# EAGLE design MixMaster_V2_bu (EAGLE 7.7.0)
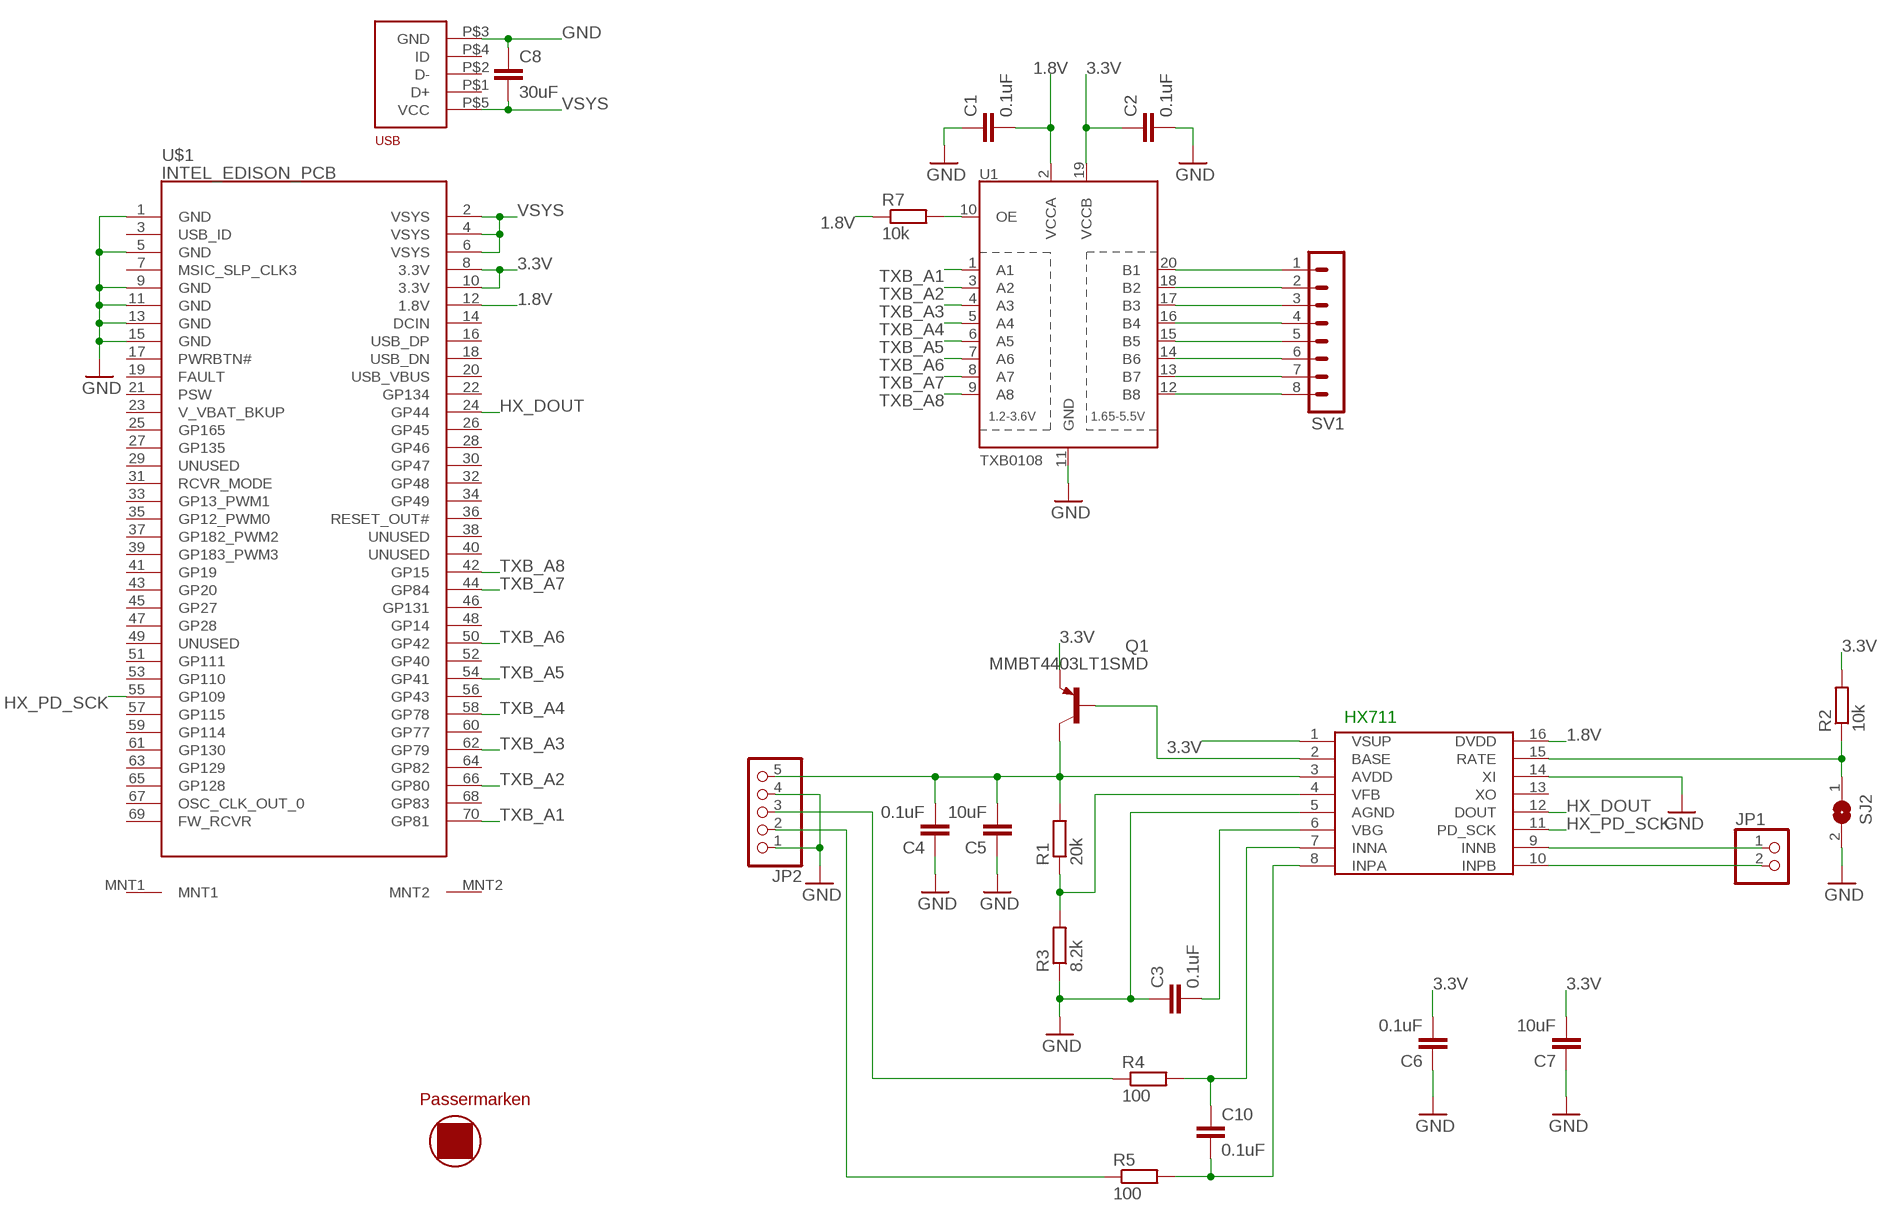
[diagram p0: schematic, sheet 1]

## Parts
C1  0.1uF  C-EUC0805  [C0805]
C2  0.1uF  C-EUC0805  [C0805]
C3  0.1uF  C-EUC0805  [C0805]
C4  0.1uF  C-EUC0805  [C0805]
C5  10uF  C-EUC0805  [C0805]
C6  0.1uF  C-EUC0805  [C0805]
C7  10uF  C-EUC0805  [C0805]
C8  30uF  C-EUC0805  [C0805]
C10  0.1uF  C-EUC0805  [C0805]
JP1  PINHD-1X2  [1X02]
JP2  PINHD-1X5  [1X05]
Q1  MMBT4403LT1SMD  [SOT23-BEC]
R1  20k  R-EU_R0805  [R0805]
R2  10k  R-EU_R0805  [R0805]
R3  8.2k  R-EU_R0805  [R0805]
R4  100  R-EU_R0805  [R0805]
R5  100  R-EU_R0805  [R0805]
R7  10k  R-EU_R0805  [R0805]
SJ2  SJ  [SJ]
SV1  MA08-1  [MA08-1]
U1  TXB0108  [TSSOP20]
U$1  INTEL_EDISON_PCB  [INTEL_EDISON]
U$2  HX711  [SO16]
U$3  USB  [USB]
U$4  PASSERMARKEN  [MASTERSUBSTRAT-MITPASSERMARKEN]

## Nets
1.8V: C1.2 R7.1 U1.2(VCCA) U$1.12(1.8V) U$2.16(DVDD)
3.3V: C2.1 C6.2 C7.2 Q1.E R2.2 U1.19(VCCB) U$1.8(3.3V) U$1.10(3.3V) U$2.1(VSUP)
GND: C1.1 C2.2 C3.1 C4.1 C5.1 C6.1 C7.1 C8.1 JP2.1 JP2.4 R3.1 SJ2.2 U1.11(GND) U$1.1(GND) U$1.5(GND) U$1.9(GND) U$1.11(GND) U$1.13(GND) U$1.15(GND) U$2.5(AGND) U$2.14(XI) U$3.P$3(GND)
HX_DOUT: U$1.24(GP44) U$2.12(DOUT)
HX_PD_SCK: U$1.55(GP109) U$2.11(PD_SCK)
N$1: R7.2 U1.10(OE)
N$2: SV1.1 U1.20(B1)
N$5: SV1.4 U1.16(B4)
N$6: SV1.5 U1.15(B5)
N$7: SV1.6 U1.14(B6)
N$8: SV1.7 U1.13(B7)
N$9: SV1.8 U1.12(B8)
N$10: C4.2 C5.2 JP2.5 Q1.C R1.2 U$2.3(AVDD)
N$11: Q1.B U$2.2(BASE)
N$12: R2.1 SJ2.1 U$2.15(RATE)
N$13: JP1.1 U$2.9(INNB)
N$14: JP1.2 U$2.10(INPB)
N$15: R1.1 R3.2 U$2.4(VFB)
N$16: JP2.2 R5.1
N$17: C3.2 U$2.6(VBG)
N$18: C10.1 R4.2 U$2.7(INNA)
N$19: C10.2 R5.2 U$2.8(INPA)
N$20: JP2.3 R4.1
N$21: SV1.2 U1.18(B2)
N$22: SV1.3 U1.17(B3)
TXB_A1: U1.1(A1) U$1.70(GP81)
TXB_A2: U1.3(A2) U$1.66(GP80)
TXB_A3: U1.4(A3) U$1.62(GP79)
TXB_A4: U1.5(A4) U$1.58(GP78)
TXB_A5: U1.6(A5) U$1.54(GP41)
TXB_A6: U1.7(A6) U$1.50(GP42)
TXB_A7: U1.8(A7) U$1.44(GP84)
TXB_A8: U1.9(A8) U$1.42(GP15)
VSYS: C8.2 U$1.2(VSYS) U$1.4(VSYS) U$1.6(VSYS) U$3.P$5(VCC)
Unconnected: U$1.3(USB_ID) U$1.7(MSIC_SLP_CLK3) U$1.14(DCIN) U$1.16(USB_DP) U$1.17(PWRBTN#) U$1.18(USB_DN) U$1.19(FAULT) U$1.20(USB_VBUS) U$1.21(PSW) U$1.22(GP134) U$1.23(V_VBAT_BKUP) U$1.25(GP165) U$1.26(GP45) U$1.27(GP135) U$1.28(GP46) U$1.29(UNUSED) U$1.30(GP47) U$1.31(RCVR_MODE) U$1.32(GP48) U$1.33(GP13_PWM1) U$1.34(GP49) U$1.35(GP12_PWM0) U$1.36(RESET_OUT#) U$1.37(GP182_PWM2) U$1.38(UNUSED) U$1.39(GP183_PWM3) U$1.40(UNUSED) U$1.41(GP19) U$1.43(GP20) U$1.45(GP27) U$1.46(GP131) U$1.47(GP28) U$1.48(GP14) U$1.49(UNUSED) U$1.51(GP111) U$1.52(GP40) U$1.53(GP110) U$1.56(GP43) U$1.57(GP115) U$1.59(GP114) U$1.60(GP77) U$1.61(GP130) U$1.63(GP129) U$1.64(GP82) U$1.65(GP128) U$1.67(OSC_CLK_OUT_0) U$1.68(GP83) U$1.69(FW_RCVR) U$1.MNT1 U$1.MNT2 U$2.13(XO) U$3.P$1(D+) U$3.P$2(D-) U$3.P$4(ID)

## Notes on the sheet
- HX711

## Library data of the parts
C1-C8 C10 = rcl:C-EU: CAPACITOR, European symbol
JP1 = pinhead:PINHD-1X2: PIN HEADER
JP2 = pinhead:PINHD-1X5: PIN HEADER
Q1 = transistor-pnp:MMBT4403*: PNP Transistror
R1-R5 R7 = rcl:R-EU_: RESISTOR, European symbol
SJ2 = jumper:SJ: SMD solder JUMPER
SV1 = con-lstb:MA08-1: PIN HEADER; OC_FARNELL: unknown; OC_NEWARK: unknown
U1 = TXB0108:TXB0108: 8-Bit Bi-Directional Level Shifter 1.2V-3.6V (VCCA) to 1.65V-5.5V (VCCB) bi-directional level shifter with auto direction sensing. Max data rate - VCCA 1.8V: 20Mbps (50ns), VCCA 3.3V: 100Mbps (10ns) Digikey: 296-21527-1-ND; AVAILABILITY: Unavailable; DESCRIPTION: 8-Bit Bidirectional Voltage-Level Translator with Auto Direction Sensing and +/-15-kV ESD Protect; MF: Texas Instruments; MP: TXB0108; PACKAGE: None; PRICE: None
U$1 = e14_Intel_Edison_RevA:INTEL_EDISON_PCB: Intel Edison Compute Module. Ideal for creating your own PCB to host an Edison. Created for www.element14.com by Dave of Young Circuit Designs. Note: 70-pin connector on the Edison is a 1.5mm-tall Hirose plug DF40C-70DP-0.4V(51) Mating Hirose receptacle connectors of varying heights include the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
U$2 = HX711:HX711
U$3 = USB_Buchse:USB
U$4 = lmhs:PASSERMARKEN

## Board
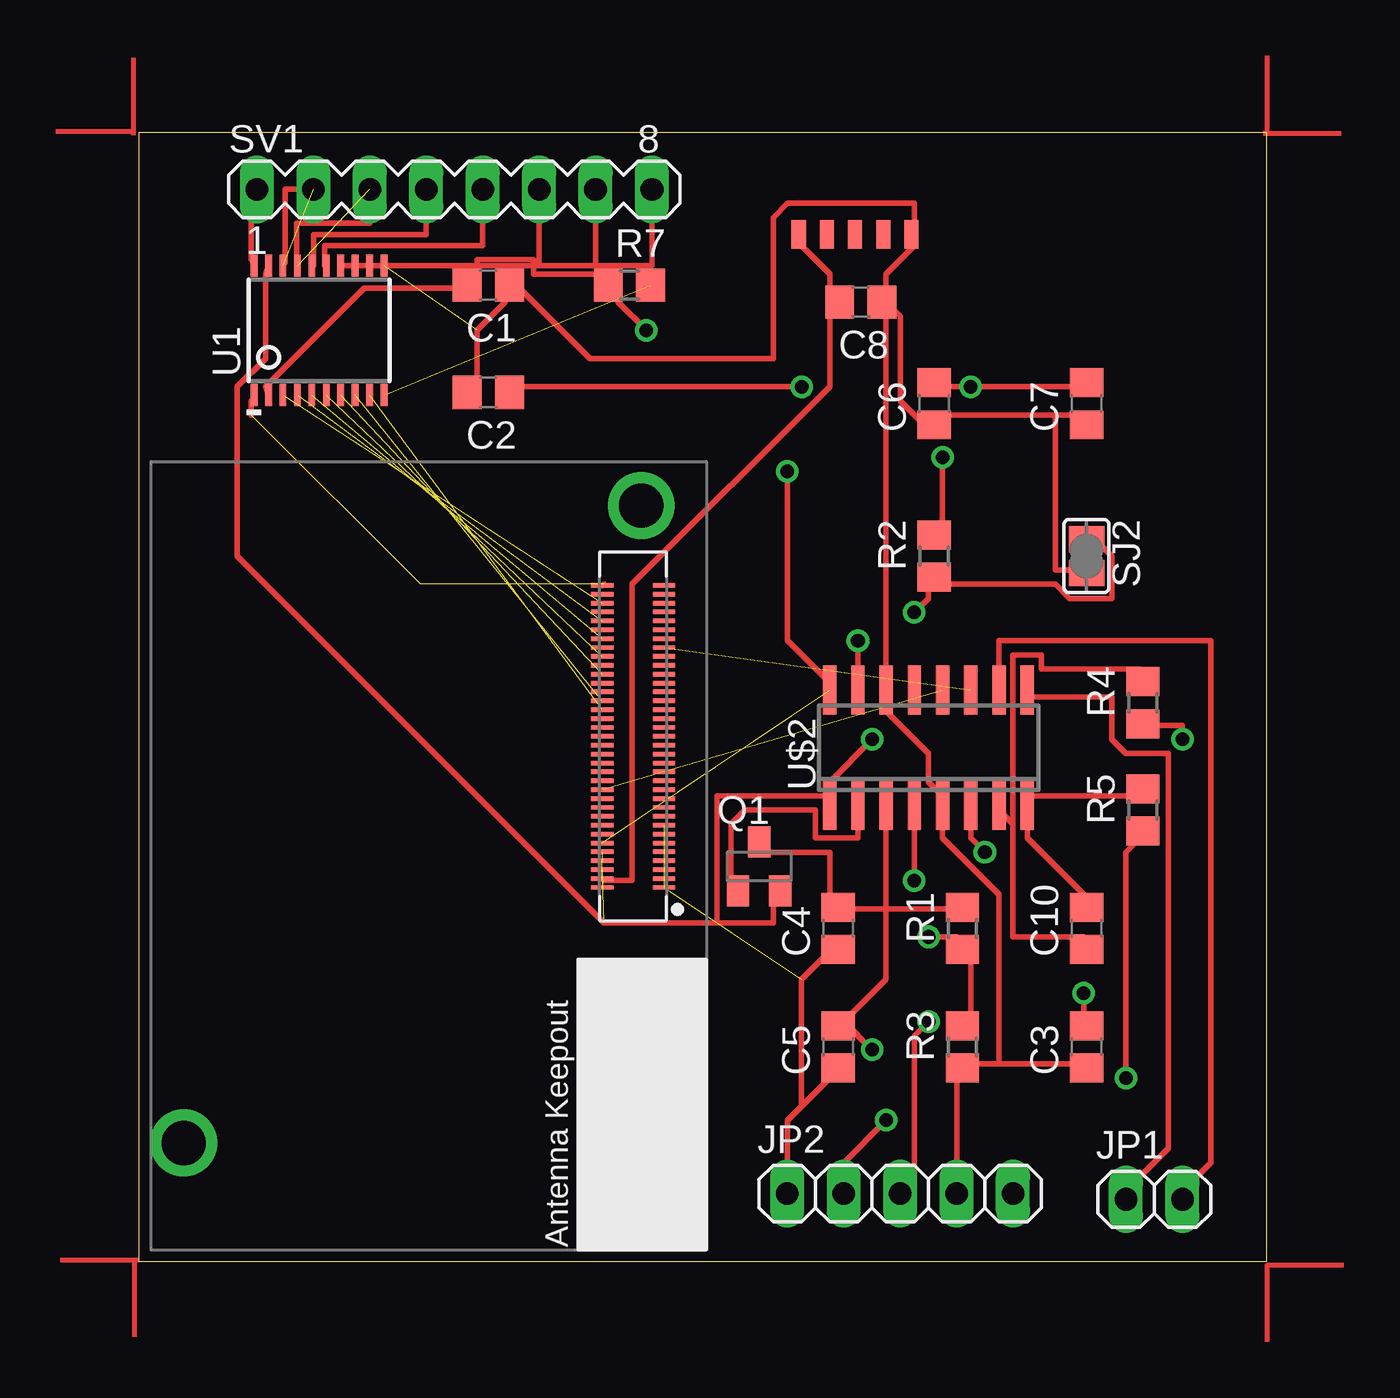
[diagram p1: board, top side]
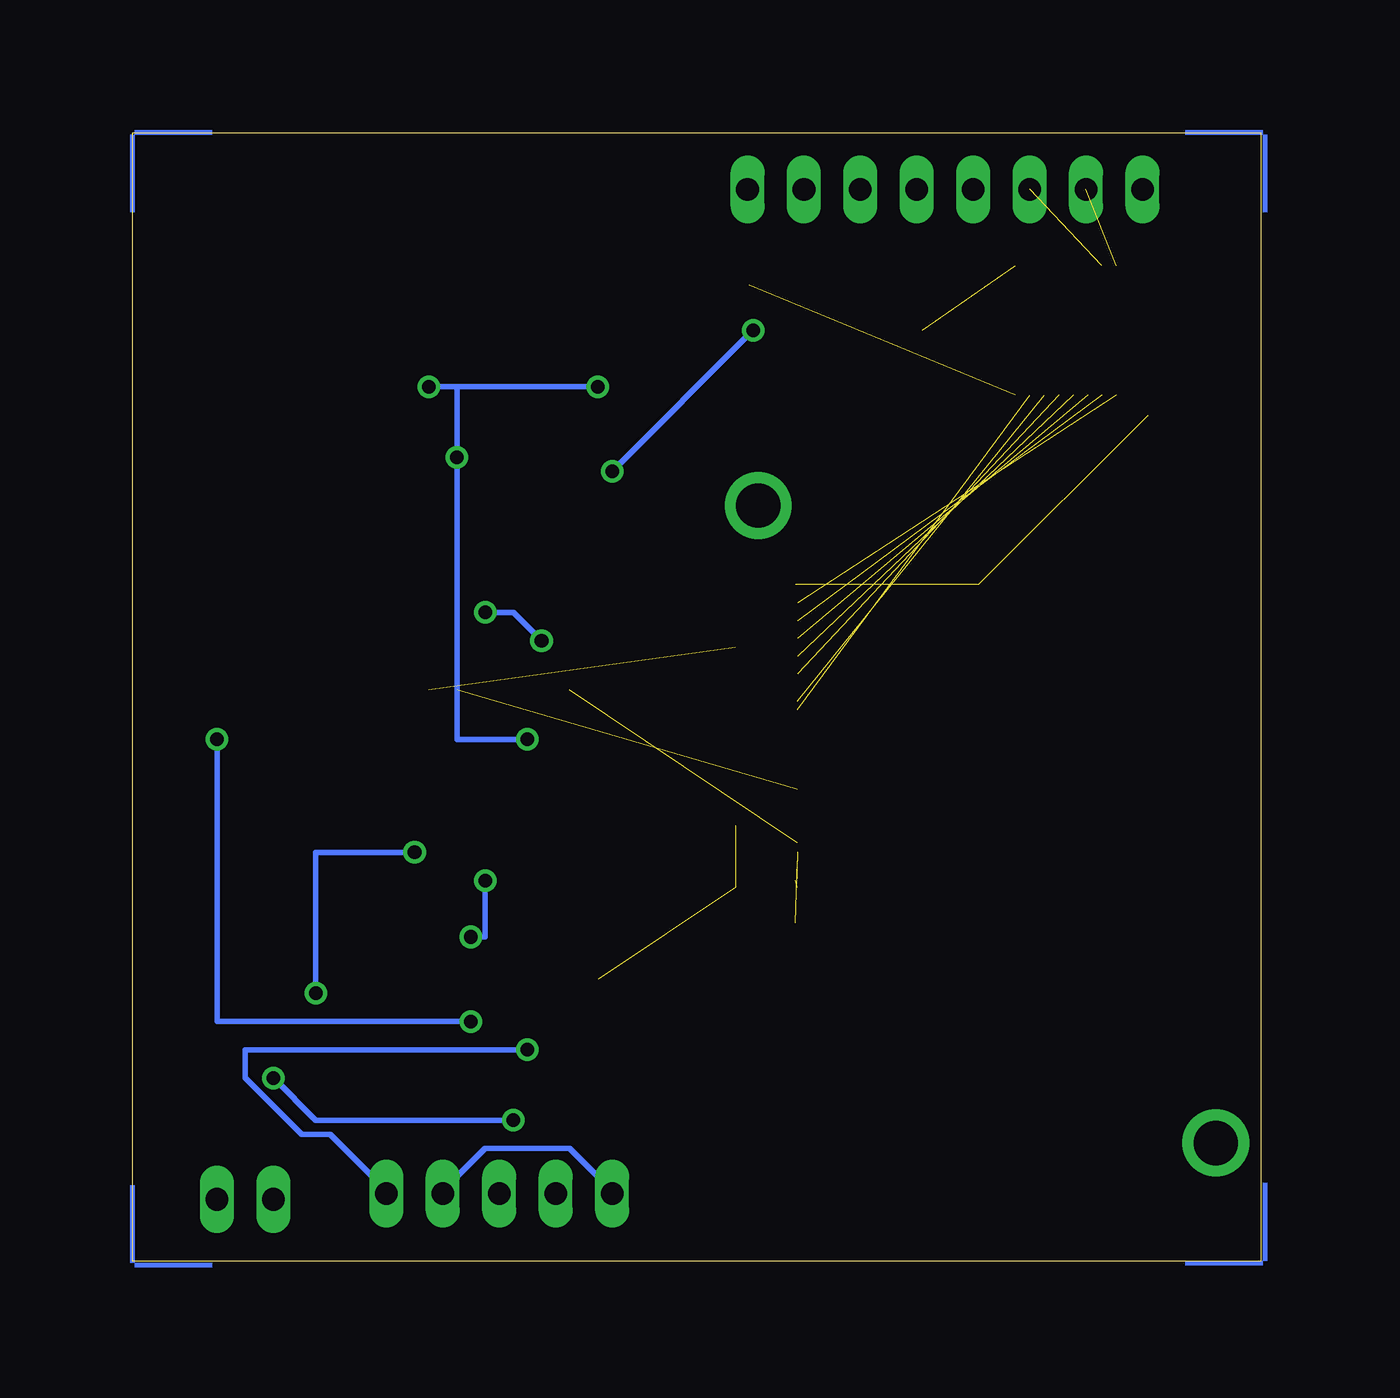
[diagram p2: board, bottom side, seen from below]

Size 50.8 x 50.8 mm. Coordinates in mm from the lower left corner, seen from the top.
Outline: 0,0 50.8,0 50.8,50.8 0,50.8 0,0
Copper layers (1*16): Top 0.035mm / dielectric 1.5mm / Bottom 0.035mm
Design rules "default": minimum track width 10mil, minimum drill 24mil, track to track 8mil, track to pad 8mil, pad to pad 8mil, via to via 8mil, smd to smd 8mil, copper to edge 40mil, drill to drill 8mil, minimum pad ring 10mil, minimum via ring 8mil, stop-mask expansion 4mil, vias tented up to drill 0mil, thermal gap 10mil

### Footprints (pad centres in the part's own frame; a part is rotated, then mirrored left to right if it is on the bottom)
C0805 = smd 1.3 x 1.5: 1 -0.95,0; 2 0.95,0
1X02 = drill 1.016 long: 1 -1.27,0; 2 1.27,0
1X05 = drill 1.016 long: 1 -5.08,0; 2 -2.54,0; 3 0,0; 4 2.54,0; 5 5.08,0
SOT23-BEC = smd 1 x 1.4: B -0.95,-1.1; C 0,1.1; E 0.95,-1.1
R0805 = smd 1.3 x 1.5: 1 -0.95,0; 2 0.95,0
SJ = smd 1.168 x 1.6: 1 -0.762,0; 2 0.762,0
MA08-1 = drill 1.016 long: 1 -8.89,0; 2 -6.35,0; 3 -3.81,0; 4 -1.27,0; 5 1.27,0; 6 3.81,0; 7 6.35,0; 8 8.89,0
TSSOP20 = smd 0.305 x 0.991: 1 -2.925,-2.918; 2 -2.275,-2.918; 3 -1.625,-2.918; 4 -0.975,-2.918; 5 -0.325,-2.918; 6 0.325,-2.918; 7 0.975,-2.918; 8 1.625,-2.918; 9 2.275,-2.918; 10 2.925,-2.918; 11 2.925,2.918; 12 2.275,2.918; 13 1.625,2.918; 14 0.975,2.918; 15 0.325,2.918; 16 -0.325,2.918; 17 -0.975,2.918; 18 -1.625,2.918; 19 -2.275,2.918; 20 -2.925,2.918
INTEL_EDISON = smd 1 x 0.2: 1 21.62,11.5; 2 18.84,11.5; 3 21.62,11.9; 4 18.84,11.9; 5 21.62,12.3; 6 18.84,12.3; 7 21.62,12.7; 8 18.84,12.7; 9 21.62,13.1; 10 18.84,13.1; 11 21.62,13.5; 12 18.84,13.5; 13 21.62,13.9; 14 18.84,13.9; 15 21.62,14.3; 16 18.84,14.3; 17 21.62,14.7; 18 18.84,14.7; 19 21.62,15.1; 20 18.84,15.1; 21 21.62,15.5; 22 18.84,15.5; 23 21.62,15.9; 24 18.84,15.9; 25 21.62,16.3; 26 18.84,16.3; 27 21.62,16.7; 28 18.84,16.7; 29 21.62,17.1; 30 18.84,17.1; 31 21.62,17.5; 32 18.84,17.5; 33 21.62,17.9; 34 18.84,17.9; 35 21.62,18.3; 36 18.84,18.3; 37 21.62,18.7; 38 18.84,18.7; 39 21.62,19.1; 40 18.84,19.1; 41 21.62,19.5; 42 18.84,19.5; 43 21.62,19.9; 44 18.84,19.9; 45 21.62,20.3; 46 18.84,20.3; 47 21.62,20.7; 48 18.84,20.7; 49 21.62,21.1; 50 18.84,21.1; 51 21.62,21.5; 52 18.84,21.5; 53 21.62,21.9; 54 18.84,21.9; 55 21.62,22.3; 56 18.84,22.3; 57 21.62,22.7; 58 18.84,22.7; 59 21.62,23.1; 60 18.84,23.1; 61 21.62,23.5; 62 18.84,23.5; 63 21.62,23.9; 64 18.84,23.9; 65 21.62,24.3; 66 18.84,24.3; 67 21.62,24.7; 68 18.84,24.7; 69 21.62,25.1; 70 18.84,25.1 | drill 2: MNT1 0,0; MNT2 20.6,28.69
SO16 = smd 0.6 x 2.2: 1 -4.445,-2.6; 2 -3.175,-2.6; 3 -1.905,-2.6; 4 -0.635,-2.6; 5 0.635,-2.6; 6 1.905,-2.6; 7 3.175,-2.6; 8 4.445,-2.6; 9 4.445,2.6; 10 3.175,2.6; 11 1.905,2.6; 12 0.635,2.6; 13 -0.635,2.6; 14 -1.905,2.6; 15 -3.175,2.6; 16 -4.445,2.6
USB = smd 1.27 x 0.635: P$1 3.81,0; P$2 3.81,1.27; P$3 3.81,2.54; P$4 3.81,-1.27; P$5 3.81,-2.54

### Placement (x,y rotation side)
C1  15.75,43.94 180 top
C2  15.75,39.12 180 top
C3  42.67,9.65 90 top
C4  31.5,14.99 90 top
C5  31.5,9.65 90 top
C6  35.81,38.61 90 top
C7  42.67,38.61 90 top
C8  32.51,43.18 180 top
C10  42.67,14.99 90 top
JP1  45.72,2.79 0 top
JP2  34.29,3.05 0 top
Q1  27.94,17.78 0 top
R1  37.08,14.99 90 top
R2  35.81,31.75 90 top
R3  37.08,9.65 90 top
R4  45.21,25.15 90 top
R5  45.21,20.32 90 top
R7  22.1,43.94 0 top
SJ2  42.67,31.75 270 top
SV1  14.22,48.26 0 top
U1  8.13,41.91 0 top
U$1  2.03,5.33 0 top
U$2  35.56,23.11 0 top
U$3  32.26,50.04 270 top
U$4  not placed on the board

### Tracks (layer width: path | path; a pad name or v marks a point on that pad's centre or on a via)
1.8V  (via drill 0.61)  (1 unrouted)
  Top 0.254: U1.2 5.71,39.37 10.16,43.81 14.61,43.81 C1.2 15.24,44.45 15.24,45.09 17.78,45.09 17.78,44.45 20.95,44.45 R7.1 21.59,43.81 21.59,43.18 v22.86,41.91 | v29.21,35.56 29.21,27.94 31.11,26.04 U$2.16
  Bottom 0.254: v22.86,41.91 v29.21,35.56
3.3V  (via drill 0.61)  (2 unrouted)
  Top 0.254: v36.2,36.2 36.2,33.02 R2.2 | C6.2 36.2,39.37 v37.47,39.37 42.55,39.37 C7.2 | v29.84,39.37 17.14,39.37 C2.1 | 26.04,15.24 28.57,15.24 28.57,16.51 Q1.E | 26.04,15.24 20.95,15.24 4.45,31.75 4.45,39.37 5.71,40.64 5.71,44.45 U1.19 | 31.11,20.95 26.04,20.95 26.04,15.24 | v33.02,23.5 31.11,21.59 31.11,20.95 | 31.11,20.95 U$2.1
  Bottom 0.254: 36.2,39.37 v36.2,36.2 36.2,23.5 v33.02,23.5 | v37.47,39.37 36.2,39.37 | 36.2,39.37 v29.84,39.37
GND  (7 unrouted)
  Top 0.254: 38.73,8.89 42.55,8.89 C3.1 | 38.73,8.89 37.47,8.89 R3.1 36.83,8.26 JP2.4 | 29.84,6.99 29.21,6.35 JP2.1 | 29.84,6.99 31.11,8.26 C5.1 | 29.84,6.99 29.84,12.7 31.11,13.97 C4.1 | C2.2 15.24,39.37 15.24,41.91 16.51,43.18 16.51,43.81 C1.1 17.14,43.81 20.32,40.64 28.57,40.64 28.57,46.99 29.21,47.62 34.92,47.62 34.92,46.35 U$3.P$3 34.92,45.72 33.66,44.45 33.66,43.18 | 41.27,38.1 42.55,38.1 C7.1 | 41.27,38.1 36.2,38.1 C6.1 35.56,37.47 34.29,38.73 34.29,42.55 33.66,43.18 | 41.27,38.1 41.27,31.11 42.55,31.11 SJ2.2 | 33.66,43.18 U$2.14 33.66,24.77 35.56,22.86 35.56,21.59 36.2,20.95 U$2.5 36.2,19.05 38.73,16.51 38.73,8.89 | 33.66,43.18 C8.1
  Bottom 0.254: JP2.4 36.83,3.17 34.92,5.08 31.11,5.08 29.21,3.17 JP2.1
HX_DOUT  (1 unrouted)
HX_PD_SCK  (1 unrouted)
N$1  (1 unrouted)
N$2
  Top 0.254: U1.20 5.08,45.09 5.08,48.26 SV1.1
N$5
  Top 0.254: U1.16 7.87,44.83 7.87,46.23 12.95,46.23 SV1.4
N$6
  Top 0.254: U1.15 8.38,44.83 8.38,45.72 15.49,45.72 SV1.5
N$7
  Top 0.254: U1.14 18.03,44.83 SV1.6
N$8
  Top 0.254: U1.13 20.57,44.83 SV1.7
N$9
  Top 0.254: U1.12 23.11,44.83 SV1.8
N$10  (via drill 0.61)
  Top 0.254: Q1.C 27.94,18.41 31.11,18.41 31.11,16.51 C4.2 31.75,15.88 33.66,15.88 | 31.75,10.79 33.66,12.7 33.66,15.88 | U$2.3 33.66,15.88 | 33.66,15.88 36.83,15.88 R1.2 | 31.75,10.79 v33.02,9.53 | 31.75,10.79 C5.2
  Bottom 0.254: v33.02,9.53 45.72,9.53 45.72,8.26 43.18,5.71 41.91,5.71 39.37,3.17 JP2.5
N$11
  Top 0.254: U$2.2 32.38,19.05 30.48,19.05 30.48,20.32 27.3,20.32 26.67,19.68 26.67,17.14 Q1.B
N$12  (via drill 0.61)
  Top 0.254: SJ2.1 43.18,32.38 43.81,31.75 43.81,29.84 41.91,29.84 41.27,30.48 36.2,30.48 R2.1 35.56,30.48 35.56,29.84 v34.92,29.21 | v32.38,27.94 U$2.15
  Bottom 0.254: v32.38,27.94 33.66,29.21 v34.92,29.21
N$13
  Top 0.254: U$2.9 40.01,25.4 43.81,25.4 43.81,23.5 44.45,22.86 46.35,22.86 46.35,5.08 44.45,3.17 JP1.1
N$14
  Top 0.254: U$2.10 38.73,27.94 48.26,27.94 48.26,4.45 46.99,3.17 JP1.2
N$15  (via drill 0.61)
  Top 0.254: R3.2 37.47,10.79 37.47,13.97 R1.1 36.83,14.61 v35.56,14.61 | v34.92,17.14 U$2.4
  Bottom 0.254: v34.92,17.14 34.92,14.61 v35.56,14.61
N$16  (via drill 0.61)
  Top 0.254: v44.45,8.26 44.45,18.41 45.09,19.05 R5.1 | v33.66,6.35 31.75,4.45 JP2.2
  Bottom 0.254: v44.45,8.26 42.55,6.35 v33.66,6.35
N$17  (via drill 0.61)
  Top 0.254: v42.55,12.06 42.55,10.79 C3.2 | v38.1,18.41 37.47,19.05 U$2.6
  Bottom 0.254: v42.55,12.06 42.55,18.41 v38.1,18.41
N$18
  Top 0.254: 39.37,19.68 39.37,14.61 42.55,14.61 C10.1 | 39.37,19.68 38.73,20.32 U$2.7 | 39.37,19.68 39.37,27.3 40.64,27.3 40.64,26.67 45.09,26.67 R4.2
N$19
  Top 0.254: C10.2 42.55,16.51 40.01,19.05 U$2.8 40.01,20.95 45.09,20.95 R5.2
N$20  (via drill 0.61)
  Top 0.254: v46.99,23.5 46.99,24.13 45.72,24.13 R4.1 | v35.56,10.79 34.92,10.16 34.92,3.81 34.29,3.17 JP2.3
  Bottom 0.254: v46.99,23.5 46.99,10.79 v35.56,10.79
N$21  (1 unrouted)
  Top 0.254: 6.6,44.96 6.6,48.26 SV1.2
N$22  (1 unrouted)
  Top 0.254: 7.11,44.96 7.11,46.74 10.41,46.74 SV1.3
TXB_A1  (2 unrouted)
  Top 0.254: 5.08,38.1 5.08,38.73 U1.1 | 20.95,30.48 U$1.70
TXB_A2  (1 unrouted)
TXB_A3  (1 unrouted)
TXB_A4  (1 unrouted)
TXB_A5  (1 unrouted)
TXB_A6  (1 unrouted)
TXB_A7  (1 unrouted)
TXB_A8  (1 unrouted)
VSYS  (2 unrouted)
  Top 0.254: 31.11,43.18 31.11,39.37 22.23,30.48 22.23,17.14 20.95,17.14 U$1.4 | 31.11,43.18 31.11,44.45 29.84,45.72 U$3.P$5 | 31.11,43.18 C8.2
